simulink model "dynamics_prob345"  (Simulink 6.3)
settings: Solver=ode3  StartTime=start_time  StopTime=stop_time  FixedStep=time_step  RelTol=1e-3
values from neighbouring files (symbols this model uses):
  ang_meas_var = 0.001    [dynamics_prob6_script.m]
  ang_proc_var = 0.001    [dynamics_prob6_script.m]
  pos_meas_var = 0.005    [dynamics_prob6_script.m]
  pos_proc_var = 0.01    [dynamics_prob6_script.m]

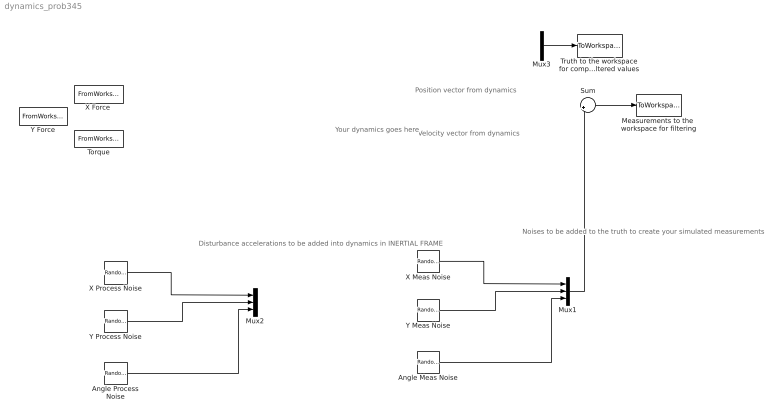
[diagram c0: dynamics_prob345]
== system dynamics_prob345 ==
  note: Position vector from dynamics
  note: Velocity vector from dynamics
  note: Disturbance accelerations to be added into dynamics in INERTIAL FRAME
  note: Noises to be added to the truth to create your simulated measurements
  note: Your dynamics goes here
  Angle Meas Noise : RandomNumber  Variance=ang_meas_var  SampleTime=0
  Angle Process Noise : RandomNumber  Variance=ang_proc_var  SampleTime=0
  Measurements to the  workspace for filtering : ToWorkspace  VariableName=meas  SampleTime=-1  SaveFormat=Structure
  Mux1 : Mux  Inputs=3
  Mux2 : Mux  Inputs=3
  Mux3 : Mux  Inputs=2
  Sum : Sum  Inputs=|++
  Torque : FromWorkspace  VariableName=torque  SampleTime=0.01  Interpolate=off  OutputAfterFinalValue=Holding final value
  Truth to the workspace for comparison with filtered values : ToWorkspace  VariableName=truth  SampleTime=-1  SaveFormat=Structure
  "X Force " : FromWorkspace  VariableName=x_force  SampleTime=0.01  Interpolate=off  OutputAfterFinalValue=Holding final value
  X Meas Noise : RandomNumber  Variance=pos_meas_var  SampleTime=0
  X Process Noise : RandomNumber  Variance=pos_proc_var  SampleTime=0
  Y Force : FromWorkspace  VariableName=y_force  SampleTime=0.01  Interpolate=off  OutputAfterFinalValue=Holding final value
  Y Meas Noise : RandomNumber  Variance=pos_meas_var  SampleTime=0
  Y Process Noise : RandomNumber  Variance=pos_proc_var  SampleTime=0
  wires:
  "X Force "/1 -> ?
  Y Force/1 -> ?
  Torque/1 -> ?
  Mux2/1 -> ?
  X Process Noise/1 -> Mux2/1
  Y Process Noise/1 -> Mux2/2
  Angle Process Noise/1 -> Mux2/3
  X Meas Noise/1 -> Mux1/1
  Y Meas Noise/1 -> Mux1/2
  Angle Meas Noise/1 -> Mux1/3
  ? -> Sum/1, Mux3/1
  Mux1/1 -> Sum/2
  Sum/1 -> Measurements to the  workspace for filtering/1
  ? -> Mux3/2
  Mux3/1 -> Truth to the workspace for comparison with filtered values/1
